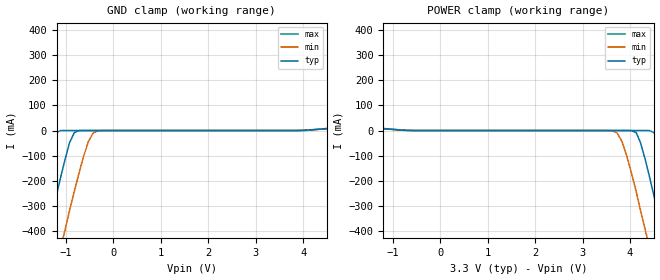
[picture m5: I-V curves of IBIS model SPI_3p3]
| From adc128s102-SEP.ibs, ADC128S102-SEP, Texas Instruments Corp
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|   Model SPI_3p3
[Model]  SPI_3p3
Model_type Input
Vinl = 0
Vinh = 3.3
C_comp   100.8fF   99.7fF   101.6fF
[Temperature Range]   25.0000   105.00   -40.00
[Voltage Range]   3.3000V   3.000V   3.60V
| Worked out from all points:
|   GND clamp passes 1 mA (typ) near -0.73 V on its own axis
|   POWER clamp passes 1 mA (typ) near -0.71 V on its own axis
[Power Clamp]
|Voltage   I(typ)   I(min)   I(max)
-3.3V     626mA      599mA      665mA
-2.71V    393mA      401mA      389mA
-1.82V    60.9mA     116mA      21.3mA
-1.32V    9.53mA     9.06mA     10.5mA
3.63V     -280pA     -1.06mA    -7.03pA
3.83V     -344nA     -44mA      -7.93pA
4.13V     -8.16mA    -242mA     -281pA
4.32V     -115mA     -394mA     -2.67uA
4.42V     -191mA     -472mA     -257uA
4.72V     -440mA     -710mA     -144mA
5.02V     -698mA     -952mA     -411mA
6.6V      -2.11A     -2.26A     -1.92A
[Gnd Clamp]
|Voltage   I(typ)   I(min)   I(max)
-3.3V     -2.11A     -2.26A     -1.92A
-1.72V    -698mA     -952mA     -411mA
-1.42V    -440mA     -710mA     -144mA
-1.12V    -191mA     -472mA     -257uA
-1.02V    -115mA     -394mA     -2.67uA
-825mV    -8.16mA    -242mA     -281pA
-528mV    -344nA     -44mA      -7.93pA
-330mV    -280pA     -1.06mA    -7.03pA
4.62V     9.53mA     9.06mA     10.5mA
5.12V     60.9mA     116mA      21.3mA
6.01V     393mA      401mA      389mA
6.6V      626mA      599mA      665mA
